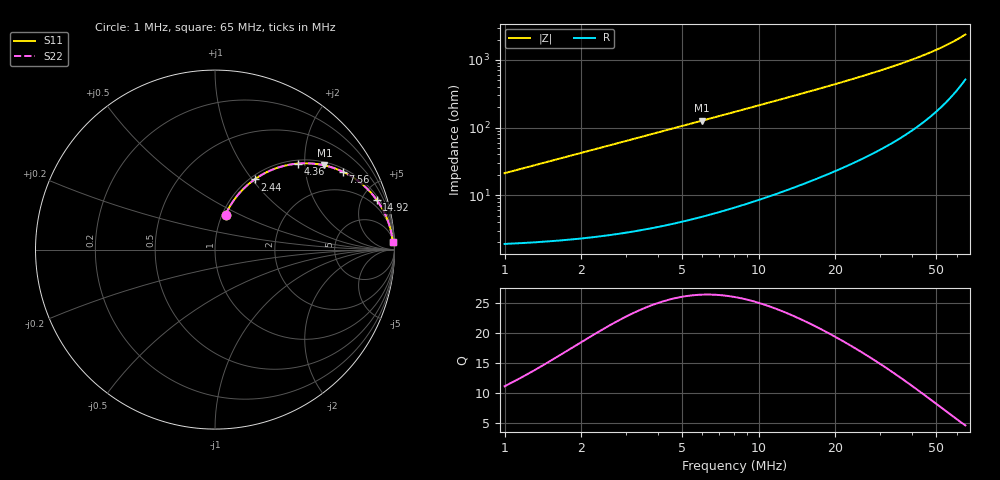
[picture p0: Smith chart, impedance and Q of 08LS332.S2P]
! Coilcraft 0805LS-332 Chip Inductor
! 18 September 2002
# MHZ S MA R 50
!Freq  MagS11  AngS11  MagS21  AngS21  MagS12  AngS12  MagS22  AngS22
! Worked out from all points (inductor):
!   401 points, 1 MHz to 65 MHz, reference 50 ohm
!   read as one part in series: L = 3.35 uH near 1.32 MHz
!   highest Q = 26.4 at 5.96 MHz (marker M1), where L = 3.36 uH
!   S11 on the Smith chart (normalised r, x): 1 MHz: 1.04, +0.42; 2.44 MHz: 1.05, +1.03; 4.36 MHz: 1.07, +1.84; 7.56 MHz: 1.12, +3.20; 14.92 MHz: 1.29, +6.42; 65 MHz: 11, +46
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1  0.2031 73.2  0.9611 -11.7  0.9611 -11.7  0.2031 73.2
1.32  0.2635 70.6  0.9458 -15.2  0.9458 -15.2  0.2635 70.6
1.48  0.2926 69.2  0.937 -17.0  0.937 -17.0  0.2926 69.2
1.8  0.3482 66.3  0.9174 -20.3  0.9174 -20.3  0.3482 66.3
2.12  0.4003 63.4  0.8956 -23.6  0.8956 -23.6  0.4003 63.4
2.44  0.4487 60.6  0.8722 -26.6  0.8722 -26.6  0.4487 60.6
3.24  0.5532 54.0  0.8098 -33.6  0.8098 -33.6  0.5532 54.0
3.72  0.6053 50.4  0.7716 -37.2  0.7716 -37.2  0.6053 50.4
4.36  0.6641 46.2  0.722 -41.6  0.722 -41.6  0.6641 46.2
5.16  0.723 41.5  0.6637 -46.3  0.6637 -46.3  0.723 41.5
5.96  0.7691 37.6  0.6107 -50.2  0.6107 -50.2  0.7691 37.6
7.56  0.8339 31.4  0.5209 -56.4  0.5209 -56.4  0.8339 31.4
9.48  0.8819 25.9  0.4379 -61.8  0.4379 -61.8  0.8819 25.9
11.72  0.9155 21.4  0.3659 -66.2  0.3659 -66.2  0.9155 21.4
14.92  0.9428 17.0  0.2934 -70.4  0.2934 -70.4  0.9428 17.0
18.28  0.9588 13.9  0.2407 -73.3  0.2407 -73.3  0.9588 13.9
22.44  0.9702 11.2  0.1948 -75.6  0.1948 -75.6  0.9702 11.2
27.24  0.9777 9.0  0.1575 -77.4  0.1575 -77.4  0.9777 9.0
33  0.9829 7.2  0.1257 -78.6  0.1257 -78.6  0.9829 7.2
43.72  0.9877 4.9  0.08634 -79.3  0.08634 -79.3  0.9877 4.9
54.44  0.9896 3.4  0.06033 -78.4  0.06033 -78.4  0.9896 3.4
65  0.9902 2.3  0.04162 -75.2  0.04162 -75.2  0.9902 2.3
